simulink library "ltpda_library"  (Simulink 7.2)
settings: Solver=ode45  SolverMode=SingleTasking  StartTime=0.0  StopTime=10.0  RelTol=1e-3
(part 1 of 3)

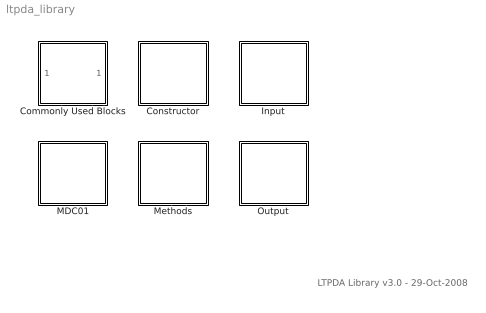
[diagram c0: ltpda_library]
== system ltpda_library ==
  note: LTPDA Library v3.0 - 29-Oct-2008
  Commonly Used Blocks : Subsystem
  Constructor : Subsystem  Tag=subsystem  AncestorBlock=libraryBase/SubSystName
  Input : Subsystem
  MDC01 : Subsystem  Tag=subsystem  AncestorBlock=libraryBase/SubSystName
  Methods : Subsystem  Tag=subsystem  AncestorBlock=libraryBase/SubSystName
  Output : Subsystem

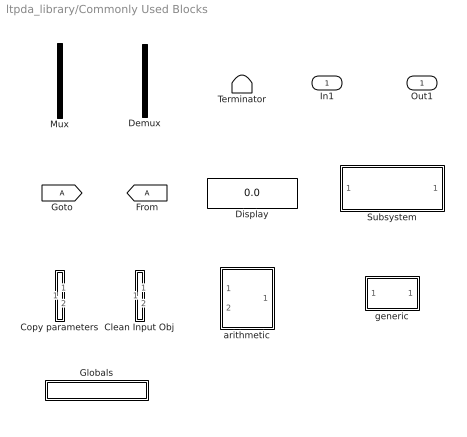
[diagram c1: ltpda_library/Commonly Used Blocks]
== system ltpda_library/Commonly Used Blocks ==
  In1 : Inport  OutDataType=sfix(16)  OutScaling=2^0
  Clean Input Obj : Subsystem
  Copy parameters : Subsystem
  Demux : Demux  Tag=demux  Outputs=2
  Display : Display
  Globals : Subsystem  Tag=globals
  Mux : Mux  Tag=mux  Inputs=2
  Subsystem : Subsystem
  Terminator : Terminator
  arithmetic : Subsystem  Tag=arithmetic
  generic : Subsystem  Tag=function
  Out1 : Outport  OutDataType=sfix(16)  OutScaling=2^0

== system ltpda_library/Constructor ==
  ltpda_getAOsInTimeSpan : Subsystem  Tag=function  AncestorBlock=libraryBase/function

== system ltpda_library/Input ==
  Object from list : Subsystem  Tag=input

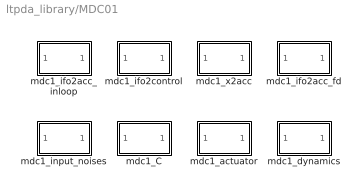
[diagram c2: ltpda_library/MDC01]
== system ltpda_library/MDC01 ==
  mdc1_C : Subsystem  Tag=function  AncestorBlock=libraryBase/function
  mdc1_actuator : Subsystem  Tag=function  AncestorBlock=libraryBase/function
  mdc1_dynamics : Subsystem  Tag=function  AncestorBlock=libraryBase/function
  mdc1_ifo2acc_fd : Subsystem  Tag=function  AncestorBlock=libraryBase/function
  mdc1_ifo2acc_inloop : Subsystem  Tag=function  AncestorBlock=libraryBase/function
  mdc1_ifo2control : Subsystem  Tag=function  AncestorBlock=libraryBase/function
  mdc1_input_noises : Subsystem  Tag=function  AncestorBlock=libraryBase/function
  mdc1_x2acc : Subsystem  Tag=function  AncestorBlock=libraryBase/function

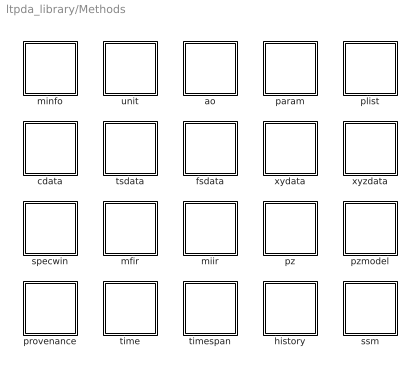
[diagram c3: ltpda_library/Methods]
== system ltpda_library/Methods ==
  ao : Subsystem  Tag=subsystem  AncestorBlock=libraryBase/SubSystName
  cdata : Subsystem  Tag=subsystem  AncestorBlock=libraryBase/SubSystName
  fsdata : Subsystem  Tag=subsystem  AncestorBlock=libraryBase/SubSystName
  history : Subsystem  Tag=subsystem  AncestorBlock=libraryBase/SubSystName
  mfir : Subsystem  Tag=subsystem  AncestorBlock=libraryBase/SubSystName
  miir : Subsystem  Tag=subsystem  AncestorBlock=libraryBase/SubSystName
  minfo : Subsystem  Tag=subsystem  AncestorBlock=libraryBase/SubSystName
  param : Subsystem  Tag=subsystem  AncestorBlock=libraryBase/SubSystName
  plist : Subsystem  Tag=subsystem  AncestorBlock=libraryBase/SubSystName
  provenance : Subsystem  Tag=subsystem  AncestorBlock=libraryBase/SubSystName
  pz : Subsystem  Tag=subsystem  AncestorBlock=libraryBase/SubSystName
  pzmodel : Subsystem  Tag=subsystem  AncestorBlock=libraryBase/SubSystName
  specwin : Subsystem  Tag=subsystem  AncestorBlock=libraryBase/SubSystName
  ssm : Subsystem  Tag=subsystem  AncestorBlock=libraryBase/SubSystName
  time : Subsystem  Tag=subsystem  AncestorBlock=libraryBase/SubSystName
  timespan : Subsystem  Tag=subsystem  AncestorBlock=libraryBase/SubSystName
  tsdata : Subsystem  Tag=subsystem  AncestorBlock=libraryBase/SubSystName
  unit : Subsystem  Tag=subsystem  AncestorBlock=libraryBase/SubSystName
  xydata : Subsystem  Tag=subsystem  AncestorBlock=libraryBase/SubSystName
  xyzdata : Subsystem  Tag=subsystem  AncestorBlock=libraryBase/SubSystName

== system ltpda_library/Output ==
  Send to output : Subsystem
  iplot : Subsystem  Tag=method ao
  plot : Subsystem  Tag=method ao
  save : Subsystem  Tag=method ao

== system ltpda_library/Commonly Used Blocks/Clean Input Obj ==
  In1 : Inport  OutDataType=sfix(16)  OutScaling=2^0
  In2 : Inport  Port=2  OutDataType=sfix(16)  OutScaling=2^0
  cleaninput : M-S-Function  FunctionName=g_cleaninput
  Out1 : Outport  OutDataType=sfix(16)  OutScaling=2^0
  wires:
  In2/1 -> cleaninput/2
  In1/1 -> cleaninput/1
  cleaninput/1 -> Out1/1

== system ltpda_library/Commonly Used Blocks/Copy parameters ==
  In1 : Inport  OutDataType=sfix(16)  OutScaling=2^0
  In2 : Inport  Port=2  OutDataType=sfix(16)  OutScaling=2^0
  copyparam : M-S-Function  FunctionName=g_copyparams
  Out1 : Outport  OutDataType=sfix(16)  OutScaling=2^0
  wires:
  copyparam/1 -> Out1/1
  In1/1 -> copyparam/1
  In2/1 -> copyparam/2

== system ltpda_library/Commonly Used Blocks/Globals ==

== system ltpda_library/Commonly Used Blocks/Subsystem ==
  In1 : Inport  OutDataType=sfix(16)  OutScaling=2^0
  Out1 : Outport  OutDataType=sfix(16)  OutScaling=2^0

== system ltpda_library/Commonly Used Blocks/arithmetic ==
  alpha : Inport  Tag=1  OutDataType=sfix(16)  OutScaling=2^0
  beta : Inport  Tag=2  Port=2  OutDataType=sfix(16)  OutScaling=2^0
  Mux : Mux  Tag=mux  Inputs=2
  arithmetic_func : M-S-Function  Tag=arithmetic  FunctionName=ltpdasim
  Out1 : Outport  OutDataType=sfix(16)  OutScaling=2^0
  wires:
  arithmetic_func/1 -> Out1/1
  Mux/1 -> arithmetic_func/1
  alpha/1 -> Mux/1
  beta/1 -> Mux/2

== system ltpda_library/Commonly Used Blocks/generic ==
  In1 : Inport  OutDataType=sfix(16)  OutScaling=2^0
  generic : M-S-Function  Tag=generic  FunctionName=ltpdasim
  Out1 : Outport  OutDataType=sfix(16)  OutScaling=2^0
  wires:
  generic/1 -> Out1/1
  In1/1 -> generic/1

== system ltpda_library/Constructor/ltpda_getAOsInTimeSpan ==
  In1 : Inport  OutDataType=sfix(16)  OutScaling=2^0
  ltpda_getAOsInTimeSpan : M-S-Function  Tag=ltpda_getAOsInTimeSpan  FunctionName=ltpdasim
  Out1 : Outport  OutDataType=sfix(16)  OutScaling=2^0
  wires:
  In1/1 -> ltpda_getAOsInTimeSpan/1
  ltpda_getAOsInTimeSpan/1 -> Out1/1

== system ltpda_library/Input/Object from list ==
  Input : Constant  Value=0  OutDataType=sfix(16)  OutScaling=2^0
  Input AO : Outport  OutDataType=sfix(16)  OutScaling=2^0
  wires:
  Input/1 -> Input AO/1

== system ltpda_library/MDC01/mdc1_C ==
  In1 : Inport  OutDataType=sfix(16)  OutScaling=2^0
  ltpda_mdc1_C : M-S-Function  Tag=ltpda_mdc1_C  FunctionName=ltpdasim
  Out1 : Outport  OutDataType=sfix(16)  OutScaling=2^0
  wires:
  In1/1 -> ltpda_mdc1_C/1
  ltpda_mdc1_C/1 -> Out1/1

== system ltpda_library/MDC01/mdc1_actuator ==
  In1 : Inport  OutDataType=sfix(16)  OutScaling=2^0
  ltpda_mdc1_actuator : M-S-Function  Tag=ltpda_mdc1_actuator  FunctionName=ltpdasim
  Out1 : Outport  OutDataType=sfix(16)  OutScaling=2^0
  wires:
  In1/1 -> ltpda_mdc1_actuator/1
  ltpda_mdc1_actuator/1 -> Out1/1

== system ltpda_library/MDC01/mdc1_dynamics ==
  In1 : Inport  OutDataType=sfix(16)  OutScaling=2^0
  ltpda_mdc1_dynamics : M-S-Function  Tag=ltpda_mdc1_dynamics  FunctionName=ltpdasim
  Out1 : Outport  OutDataType=sfix(16)  OutScaling=2^0
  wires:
  In1/1 -> ltpda_mdc1_dynamics/1
  ltpda_mdc1_dynamics/1 -> Out1/1

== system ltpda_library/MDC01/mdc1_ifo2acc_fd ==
  In1 : Inport  OutDataType=sfix(16)  OutScaling=2^0
  ltpda_mdc1_ifo2acc_fd : M-S-Function  Tag=ltpda_mdc1_ifo2acc_fd  FunctionName=ltpdasim
  Out1 : Outport  OutDataType=sfix(16)  OutScaling=2^0
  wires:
  In1/1 -> ltpda_mdc1_ifo2acc_fd/1
  ltpda_mdc1_ifo2acc_fd/1 -> Out1/1

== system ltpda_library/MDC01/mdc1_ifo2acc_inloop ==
  In1 : Inport  OutDataType=sfix(16)  OutScaling=2^0
  ltpda_mdc1_ifo2acc_inloop : M-S-Function  Tag=ltpda_mdc1_ifo2acc_inloop  FunctionName=ltpdasim
  Out1 : Outport  OutDataType=sfix(16)  OutScaling=2^0
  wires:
  In1/1 -> ltpda_mdc1_ifo2acc_inloop/1
  ltpda_mdc1_ifo2acc_inloop/1 -> Out1/1

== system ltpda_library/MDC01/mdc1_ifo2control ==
  In1 : Inport  OutDataType=sfix(16)  OutScaling=2^0
  ltpda_mdc1_ifo2control : M-S-Function  Tag=ltpda_mdc1_ifo2control  FunctionName=ltpdasim
  Out1 : Outport  OutDataType=sfix(16)  OutScaling=2^0
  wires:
  In1/1 -> ltpda_mdc1_ifo2control/1
  ltpda_mdc1_ifo2control/1 -> Out1/1

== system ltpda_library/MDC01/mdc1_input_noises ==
  In1 : Inport  OutDataType=sfix(16)  OutScaling=2^0
  ltpda_mdc1_input_noises : M-S-Function  Tag=ltpda_mdc1_input_noises  FunctionName=ltpdasim
  Out1 : Outport  OutDataType=sfix(16)  OutScaling=2^0
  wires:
  In1/1 -> ltpda_mdc1_input_noises/1
  ltpda_mdc1_input_noises/1 -> Out1/1

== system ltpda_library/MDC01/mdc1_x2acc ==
  In1 : Inport  OutDataType=sfix(16)  OutScaling=2^0
  ltpda_mdc1_x2acc : M-S-Function  Tag=ltpda_mdc1_x2acc  FunctionName=ltpdasim
  Out1 : Outport  OutDataType=sfix(16)  OutScaling=2^0
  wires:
  In1/1 -> ltpda_mdc1_x2acc/1
  ltpda_mdc1_x2acc/1 -> Out1/1

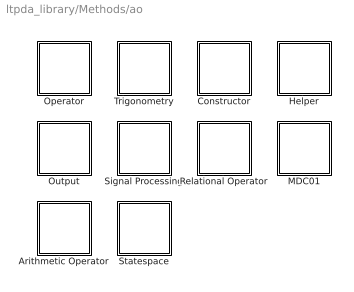
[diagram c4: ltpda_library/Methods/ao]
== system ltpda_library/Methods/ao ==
  Arithmetic Operator : Subsystem  Tag=subsystem  AncestorBlock=libraryBase/SubSystName
  Constructor : Subsystem  Tag=subsystem  AncestorBlock=libraryBase/SubSystName
  Helper : Subsystem  Tag=subsystem  AncestorBlock=libraryBase/SubSystName
  MDC01 : Subsystem  Tag=subsystem  AncestorBlock=libraryBase/SubSystName
  Operator : Subsystem  Tag=subsystem  AncestorBlock=libraryBase/SubSystName
  Output : Subsystem  Tag=subsystem  AncestorBlock=libraryBase/SubSystName
  Relational Operator : Subsystem  Tag=subsystem  AncestorBlock=libraryBase/SubSystName
  Signal Processing : Subsystem  Tag=subsystem  AncestorBlock=libraryBase/SubSystName
  Statespace : Subsystem  Tag=subsystem  AncestorBlock=libraryBase/SubSystName
  Trigonometry : Subsystem  Tag=subsystem  AncestorBlock=libraryBase/SubSystName

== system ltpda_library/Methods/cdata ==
  Constructor : Subsystem  Tag=subsystem  AncestorBlock=libraryBase/SubSystName
  Helper : Subsystem  Tag=subsystem  AncestorBlock=libraryBase/SubSystName
  Output : Subsystem  Tag=subsystem  AncestorBlock=libraryBase/SubSystName
  Relational Operator : Subsystem  Tag=subsystem  AncestorBlock=libraryBase/SubSystName

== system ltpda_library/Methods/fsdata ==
  Constructor : Subsystem  Tag=subsystem  AncestorBlock=libraryBase/SubSystName
  Helper : Subsystem  Tag=subsystem  AncestorBlock=libraryBase/SubSystName
  Output : Subsystem  Tag=subsystem  AncestorBlock=libraryBase/SubSystName
  Relational Operator : Subsystem  Tag=subsystem  AncestorBlock=libraryBase/SubSystName

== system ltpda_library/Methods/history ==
  Constructor : Subsystem  Tag=subsystem  AncestorBlock=libraryBase/SubSystName
  Helper : Subsystem  Tag=subsystem  AncestorBlock=libraryBase/SubSystName
  Output : Subsystem  Tag=subsystem  AncestorBlock=libraryBase/SubSystName
  Relational Operator : Subsystem  Tag=subsystem  AncestorBlock=libraryBase/SubSystName

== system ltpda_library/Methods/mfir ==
  Constructor : Subsystem  Tag=subsystem  AncestorBlock=libraryBase/SubSystName
  Helper : Subsystem  Tag=subsystem  AncestorBlock=libraryBase/SubSystName
  Output : Subsystem  Tag=subsystem  AncestorBlock=libraryBase/SubSystName
  Relational Operator : Subsystem  Tag=subsystem  AncestorBlock=libraryBase/SubSystName
  Signal Processing : Subsystem  Tag=subsystem  AncestorBlock=libraryBase/SubSystName
  Statespace : Subsystem  Tag=subsystem  AncestorBlock=libraryBase/SubSystName

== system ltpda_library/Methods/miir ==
  Constructor : Subsystem  Tag=subsystem  AncestorBlock=libraryBase/SubSystName
  Helper : Subsystem  Tag=subsystem  AncestorBlock=libraryBase/SubSystName
  Output : Subsystem  Tag=subsystem  AncestorBlock=libraryBase/SubSystName
  Relational Operator : Subsystem  Tag=subsystem  AncestorBlock=libraryBase/SubSystName
  Signal Processing : Subsystem  Tag=subsystem  AncestorBlock=libraryBase/SubSystName
  Statespace : Subsystem  Tag=subsystem  AncestorBlock=libraryBase/SubSystName

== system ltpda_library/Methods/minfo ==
  Constructor : Subsystem  Tag=subsystem  AncestorBlock=libraryBase/SubSystName
  Helper : Subsystem  Tag=subsystem  AncestorBlock=libraryBase/SubSystName
  Output : Subsystem  Tag=subsystem  AncestorBlock=libraryBase/SubSystName
  Relational Operator : Subsystem  Tag=subsystem  AncestorBlock=libraryBase/SubSystName

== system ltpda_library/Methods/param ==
  Constructor : Subsystem  Tag=subsystem  AncestorBlock=libraryBase/SubSystName
  Helper : Subsystem  Tag=subsystem  AncestorBlock=libraryBase/SubSystName
  Output : Subsystem  Tag=subsystem  AncestorBlock=libraryBase/SubSystName
  Relational Operator : Subsystem  Tag=subsystem  AncestorBlock=libraryBase/SubSystName

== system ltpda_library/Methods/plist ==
  Constructor : Subsystem  Tag=subsystem  AncestorBlock=libraryBase/SubSystName
  Helper : Subsystem  Tag=subsystem  AncestorBlock=libraryBase/SubSystName
  Output : Subsystem  Tag=subsystem  AncestorBlock=libraryBase/SubSystName
  Relational Operator : Subsystem  Tag=subsystem  AncestorBlock=libraryBase/SubSystName
  Signal Processing : Subsystem  Tag=subsystem  AncestorBlock=libraryBase/SubSystName

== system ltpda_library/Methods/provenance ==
  Constructor : Subsystem  Tag=subsystem  AncestorBlock=libraryBase/SubSystName
  Helper : Subsystem  Tag=subsystem  AncestorBlock=libraryBase/SubSystName
  Output : Subsystem  Tag=subsystem  AncestorBlock=libraryBase/SubSystName
  Relational Operator : Subsystem  Tag=subsystem  AncestorBlock=libraryBase/SubSystName

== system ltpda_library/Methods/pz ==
  Constructor : Subsystem  Tag=subsystem  AncestorBlock=libraryBase/SubSystName
  Helper : Subsystem  Tag=subsystem  AncestorBlock=libraryBase/SubSystName
  Output : Subsystem  Tag=subsystem  AncestorBlock=libraryBase/SubSystName
  Relational Operator : Subsystem  Tag=subsystem  AncestorBlock=libraryBase/SubSystName
  Signal Processing : Subsystem  Tag=subsystem  AncestorBlock=libraryBase/SubSystName

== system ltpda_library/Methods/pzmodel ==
  Constructor : Subsystem  Tag=subsystem  AncestorBlock=libraryBase/SubSystName
  Helper : Subsystem  Tag=subsystem  AncestorBlock=libraryBase/SubSystName
  Operator : Subsystem  Tag=subsystem  AncestorBlock=libraryBase/SubSystName
  Output : Subsystem  Tag=subsystem  AncestorBlock=libraryBase/SubSystName
  Relational Operator : Subsystem  Tag=subsystem  AncestorBlock=libraryBase/SubSystName
  Signal Processing : Subsystem  Tag=subsystem  AncestorBlock=libraryBase/SubSystName
  Statespace : Subsystem  Tag=subsystem  AncestorBlock=libraryBase/SubSystName

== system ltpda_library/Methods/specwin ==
  Constructor : Subsystem  Tag=subsystem  AncestorBlock=libraryBase/SubSystName
  Helper : Subsystem  Tag=subsystem  AncestorBlock=libraryBase/SubSystName
  Output : Subsystem  Tag=subsystem  AncestorBlock=libraryBase/SubSystName
  Relational Operator : Subsystem  Tag=subsystem  AncestorBlock=libraryBase/SubSystName

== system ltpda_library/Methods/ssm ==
  Constructor : Subsystem  Tag=subsystem  AncestorBlock=libraryBase/SubSystName
  Helper : Subsystem  Tag=subsystem  AncestorBlock=libraryBase/SubSystName
  Output : Subsystem  Tag=subsystem  AncestorBlock=libraryBase/SubSystName
  Relational Operator : Subsystem  Tag=subsystem  AncestorBlock=libraryBase/SubSystName
  STATESPACE : Subsystem  Tag=subsystem  AncestorBlock=libraryBase/SubSystName
  Statespace : Subsystem  Tag=subsystem  AncestorBlock=libraryBase/SubSystName

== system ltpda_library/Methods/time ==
  Arithmetic Operator : Subsystem  Tag=subsystem  AncestorBlock=libraryBase/SubSystName
  Constructor : Subsystem  Tag=subsystem  AncestorBlock=libraryBase/SubSystName
  Helper : Subsystem  Tag=subsystem  AncestorBlock=libraryBase/SubSystName
  Output : Subsystem  Tag=subsystem  AncestorBlock=libraryBase/SubSystName
  Relational Operator : Subsystem  Tag=subsystem  AncestorBlock=libraryBase/SubSystName

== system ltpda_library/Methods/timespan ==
  Constructor : Subsystem  Tag=subsystem  AncestorBlock=libraryBase/SubSystName
  Helper : Subsystem  Tag=subsystem  AncestorBlock=libraryBase/SubSystName
  Output : Subsystem  Tag=subsystem  AncestorBlock=libraryBase/SubSystName
  Relational Operator : Subsystem  Tag=subsystem  AncestorBlock=libraryBase/SubSystName
  Statespace : Subsystem  Tag=subsystem  AncestorBlock=libraryBase/SubSystName

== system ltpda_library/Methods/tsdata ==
  Constructor : Subsystem  Tag=subsystem  AncestorBlock=libraryBase/SubSystName
  Helper : Subsystem  Tag=subsystem  AncestorBlock=libraryBase/SubSystName
  Output : Subsystem  Tag=subsystem  AncestorBlock=libraryBase/SubSystName
  Relational Operator : Subsystem  Tag=subsystem  AncestorBlock=libraryBase/SubSystName

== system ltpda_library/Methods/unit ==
  Constructor : Subsystem  Tag=subsystem  AncestorBlock=libraryBase/SubSystName
  Helper : Subsystem  Tag=subsystem  AncestorBlock=libraryBase/SubSystName
  Output : Subsystem  Tag=subsystem  AncestorBlock=libraryBase/SubSystName
  Relational Operator : Subsystem  Tag=subsystem  AncestorBlock=libraryBase/SubSystName

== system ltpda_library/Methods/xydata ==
  Constructor : Subsystem  Tag=subsystem  AncestorBlock=libraryBase/SubSystName
  Helper : Subsystem  Tag=subsystem  AncestorBlock=libraryBase/SubSystName
  Output : Subsystem  Tag=subsystem  AncestorBlock=libraryBase/SubSystName
  Relational Operator : Subsystem  Tag=subsystem  AncestorBlock=libraryBase/SubSystName

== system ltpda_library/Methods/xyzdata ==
  Constructor : Subsystem  Tag=subsystem  AncestorBlock=libraryBase/SubSystName
  Helper : Subsystem  Tag=subsystem  AncestorBlock=libraryBase/SubSystName
  Output : Subsystem  Tag=subsystem  AncestorBlock=libraryBase/SubSystName
  Relational Operator : Subsystem  Tag=subsystem  AncestorBlock=libraryBase/SubSystName

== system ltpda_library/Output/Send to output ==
  In1 : Inport  OutDataType=sfix(16)  OutScaling=2^0
  save result : M-S-Function  FunctionName=g_saveresult
  Out1 : Outport  OutDataType=sfix(16)  OutScaling=2^0
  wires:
  In1/1 -> save result/1
  save result/1 -> Out1/1

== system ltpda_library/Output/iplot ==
  In1 : Inport  OutDataType=sfix(16)  OutScaling=2^0
  Terminator : Terminator
  iplot : M-S-Function  Tag=iplot  FunctionName=ltpdasim
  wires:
  In1/1 -> iplot/1
  iplot/1 -> Terminator/1

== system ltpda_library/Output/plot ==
  In1 : Inport  OutDataType=sfix(16)  OutScaling=2^0
  Terminator : Terminator
  plot : M-S-Function  Tag=plot  FunctionName=ltpdasim
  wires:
  In1/1 -> plot/1
  plot/1 -> Terminator/1

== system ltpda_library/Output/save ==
  In1 : Inport  OutDataType=sfix(16)  OutScaling=2^0
  Terminator : Terminator
  save : M-S-Function  Tag=save  FunctionName=ltpdasim
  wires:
  In1/1 -> save/1
  save/1 -> Terminator/1

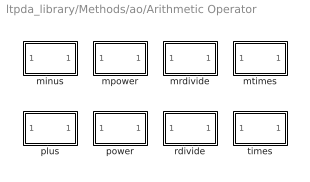
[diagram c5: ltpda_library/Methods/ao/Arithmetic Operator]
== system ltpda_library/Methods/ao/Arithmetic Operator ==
  minus : Subsystem  Tag=method ao  AncestorBlock=libraryBase/function
  mpower : Subsystem  Tag=method ao  AncestorBlock=libraryBase/function
  mrdivide : Subsystem  Tag=method ao  AncestorBlock=libraryBase/function
  mtimes : Subsystem  Tag=method ao  AncestorBlock=libraryBase/function
  plus : Subsystem  Tag=method ao  AncestorBlock=libraryBase/function
  power : Subsystem  Tag=method ao  AncestorBlock=libraryBase/function
  rdivide : Subsystem  Tag=method ao  AncestorBlock=libraryBase/function
  times : Subsystem  Tag=method ao  AncestorBlock=libraryBase/function

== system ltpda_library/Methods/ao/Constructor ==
  ao : Subsystem  Tag=method ao  AncestorBlock=libraryBase/constructor
  rebuild : Subsystem  Tag=method ao  AncestorBlock=libraryBase/constructor

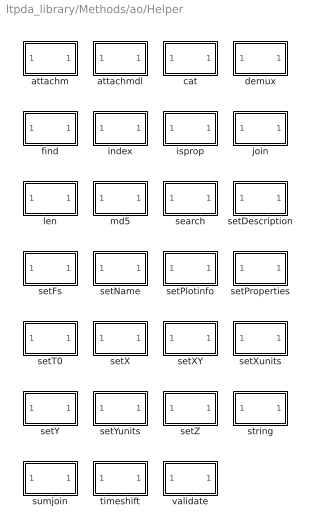
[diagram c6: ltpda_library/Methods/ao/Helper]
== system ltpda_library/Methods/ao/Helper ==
  attachm : Subsystem  Tag=method ao  AncestorBlock=libraryBase/function
  attachmdl : Subsystem  Tag=method ao  AncestorBlock=libraryBase/function
  cat : Subsystem  Tag=method ao  AncestorBlock=libraryBase/function
  demux : Subsystem  Tag=method ao  AncestorBlock=libraryBase/function
  find : Subsystem  Tag=method ao  AncestorBlock=libraryBase/function
  index : Subsystem  Tag=method ao  AncestorBlock=libraryBase/function
  isprop : Subsystem  Tag=method ao  AncestorBlock=libraryBase/function
  join : Subsystem  Tag=method ao  AncestorBlock=libraryBase/function
  len : Subsystem  Tag=method ao  AncestorBlock=libraryBase/function
  md5 : Subsystem  Tag=method ao  AncestorBlock=libraryBase/function
  search : Subsystem  Tag=method ao  AncestorBlock=libraryBase/function
  setDescription : Subsystem  Tag=method ao  AncestorBlock=libraryBase/function
  setFs : Subsystem  Tag=method ao  AncestorBlock=libraryBase/function
  setName : Subsystem  Tag=method ao  AncestorBlock=libraryBase/function
  setPlotinfo : Subsystem  Tag=method ao  AncestorBlock=libraryBase/function
  setProperties : Subsystem  Tag=method ao  AncestorBlock=libraryBase/function
  setT0 : Subsystem  Tag=method ao  AncestorBlock=libraryBase/function
  setX : Subsystem  Tag=method ao  AncestorBlock=libraryBase/function
  setXY : Subsystem  Tag=method ao  AncestorBlock=libraryBase/function
  setXunits : Subsystem  Tag=method ao  AncestorBlock=libraryBase/function
  setY : Subsystem  Tag=method ao  AncestorBlock=libraryBase/function
  setYunits : Subsystem  Tag=method ao  AncestorBlock=libraryBase/function
  setZ : Subsystem  Tag=method ao  AncestorBlock=libraryBase/function
  string : Subsystem  Tag=method ao  AncestorBlock=libraryBase/function
  sumjoin : Subsystem  Tag=method ao  AncestorBlock=libraryBase/function
  timeshift : Subsystem  Tag=method ao  AncestorBlock=libraryBase/function
  validate : Subsystem  Tag=method ao  AncestorBlock=libraryBase/function

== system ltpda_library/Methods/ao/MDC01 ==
  mdc1_ifo2acc_fd : Subsystem  Tag=method ao  AncestorBlock=libraryBase/function
  mdc1_ifo2acc_inloop : Subsystem  Tag=method ao  AncestorBlock=libraryBase/function
  mdc1_ifo2control : Subsystem  Tag=method ao  AncestorBlock=libraryBase/function
  mdc1_x2acc : Subsystem  Tag=method ao  AncestorBlock=libraryBase/function

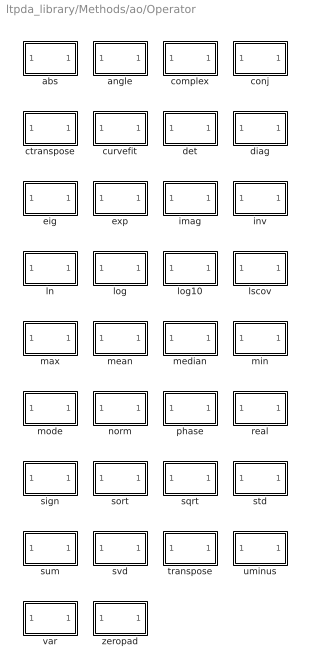
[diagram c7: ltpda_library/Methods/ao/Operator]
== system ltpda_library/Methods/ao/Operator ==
  abs : Subsystem  Tag=method ao  AncestorBlock=libraryBase/function
  angle : Subsystem  Tag=method ao  AncestorBlock=libraryBase/function
  complex : Subsystem  Tag=method ao  AncestorBlock=libraryBase/function
  conj : Subsystem  Tag=method ao  AncestorBlock=libraryBase/function
  ctranspose : Subsystem  Tag=method ao  AncestorBlock=libraryBase/function
  curvefit : Subsystem  Tag=method ao  AncestorBlock=libraryBase/function
  det : Subsystem  Tag=method ao  AncestorBlock=libraryBase/function
  diag : Subsystem  Tag=method ao  AncestorBlock=libraryBase/function
  eig : Subsystem  Tag=method ao  AncestorBlock=libraryBase/function
  exp : Subsystem  Tag=method ao  AncestorBlock=libraryBase/function
  imag : Subsystem  Tag=method ao  AncestorBlock=libraryBase/function
  inv : Subsystem  Tag=method ao  AncestorBlock=libraryBase/function
  ln : Subsystem  Tag=method ao  AncestorBlock=libraryBase/function
  log : Subsystem  Tag=method ao  AncestorBlock=libraryBase/function
  log10 : Subsystem  Tag=method ao  AncestorBlock=libraryBase/function
  lscov : Subsystem  Tag=method ao  AncestorBlock=libraryBase/function
  max : Subsystem  Tag=method ao  AncestorBlock=libraryBase/function
  mean : Subsystem  Tag=method ao  AncestorBlock=libraryBase/function
  median : Subsystem  Tag=method ao  AncestorBlock=libraryBase/function
  min : Subsystem  Tag=method ao  AncestorBlock=libraryBase/function
  mode : Subsystem  Tag=method ao  AncestorBlock=libraryBase/function
  norm : Subsystem  Tag=method ao  AncestorBlock=libraryBase/function
  phase : Subsystem  Tag=method ao  AncestorBlock=libraryBase/function
  real : Subsystem  Tag=method ao  AncestorBlock=libraryBase/function
  sign : Subsystem  Tag=method ao  AncestorBlock=libraryBase/function
  sort : Subsystem  Tag=method ao  AncestorBlock=libraryBase/function
  sqrt : Subsystem  Tag=method ao  AncestorBlock=libraryBase/function
  std : Subsystem  Tag=method ao  AncestorBlock=libraryBase/function
  sum : Subsystem  Tag=method ao  AncestorBlock=libraryBase/function
  svd : Subsystem  Tag=method ao  AncestorBlock=libraryBase/function
  transpose : Subsystem  Tag=method ao  AncestorBlock=libraryBase/function
  uminus : Subsystem  Tag=method ao  AncestorBlock=libraryBase/function
  var : Subsystem  Tag=method ao  AncestorBlock=libraryBase/function
  zeropad : Subsystem  Tag=method ao  AncestorBlock=libraryBase/function

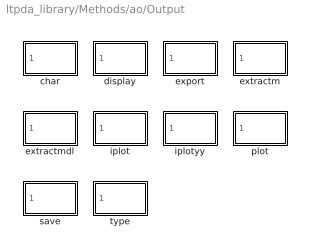
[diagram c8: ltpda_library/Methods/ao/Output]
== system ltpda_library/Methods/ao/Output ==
  char : Subsystem  Tag=method ao  AncestorBlock=libraryBase/output
  display : Subsystem  Tag=method ao  AncestorBlock=libraryBase/output
  export : Subsystem  Tag=method ao  AncestorBlock=libraryBase/output
  extractm : Subsystem  Tag=method ao  AncestorBlock=libraryBase/output
  extractmdl : Subsystem  Tag=method ao  AncestorBlock=libraryBase/output
  iplot : Subsystem  Tag=method ao  AncestorBlock=libraryBase/output
  iplotyy : Subsystem  Tag=method ao  AncestorBlock=libraryBase/output
  plot : Subsystem  Tag=method ao  AncestorBlock=libraryBase/output
  save : Subsystem  Tag=method ao  AncestorBlock=libraryBase/output
  type : Subsystem  Tag=method ao  AncestorBlock=libraryBase/output

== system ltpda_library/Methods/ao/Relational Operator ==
  eq : Subsystem  Tag=method ao  AncestorBlock=libraryBase/function
  ge : Subsystem  Tag=method ao  AncestorBlock=libraryBase/function
  gt : Subsystem  Tag=method ao  AncestorBlock=libraryBase/function
  le : Subsystem  Tag=method ao  AncestorBlock=libraryBase/function
  lt : Subsystem  Tag=method ao  AncestorBlock=libraryBase/function
  ne : Subsystem  Tag=method ao  AncestorBlock=libraryBase/function

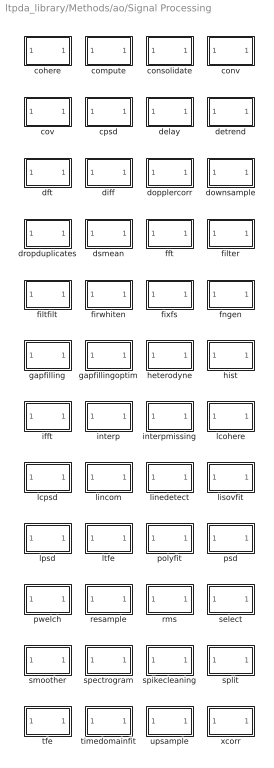
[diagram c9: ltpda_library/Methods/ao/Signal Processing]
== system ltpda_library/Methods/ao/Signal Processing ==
  cohere : Subsystem  Tag=method ao  AncestorBlock=libraryBase/function
  compute : Subsystem  Tag=method ao  AncestorBlock=libraryBase/function
  consolidate : Subsystem  Tag=method ao  AncestorBlock=libraryBase/function
  conv : Subsystem  Tag=method ao  AncestorBlock=libraryBase/function
  cov : Subsystem  Tag=method ao  AncestorBlock=libraryBase/function
  cpsd : Subsystem  Tag=method ao  AncestorBlock=libraryBase/function
  delay : Subsystem  Tag=method ao  AncestorBlock=libraryBase/function
  detrend : Subsystem  Tag=method ao  AncestorBlock=libraryBase/function
  dft : Subsystem  Tag=method ao  AncestorBlock=libraryBase/function
  diff : Subsystem  Tag=method ao  AncestorBlock=libraryBase/function
  dopplercorr : Subsystem  Tag=method ao  AncestorBlock=libraryBase/function
  downsample : Subsystem  Tag=method ao  AncestorBlock=libraryBase/function
  dropduplicates : Subsystem  Tag=method ao  AncestorBlock=libraryBase/function
  dsmean : Subsystem  Tag=method ao  AncestorBlock=libraryBase/function
  fft : Subsystem  Tag=method ao  AncestorBlock=libraryBase/function
  filter : Subsystem  Tag=method ao  AncestorBlock=libraryBase/function
  filtfilt : Subsystem  Tag=method ao  AncestorBlock=libraryBase/function
  firwhiten : Subsystem  Tag=method ao  AncestorBlock=libraryBase/function
  fixfs : Subsystem  Tag=method ao  AncestorBlock=libraryBase/function
  fngen : Subsystem  Tag=method ao  AncestorBlock=libraryBase/function
  gapfilling : Subsystem  Tag=method ao  AncestorBlock=libraryBase/function
  gapfillingoptim : Subsystem  Tag=method ao  AncestorBlock=libraryBase/function
  heterodyne : Subsystem  Tag=method ao  AncestorBlock=libraryBase/function
  hist : Subsystem  Tag=method ao  AncestorBlock=libraryBase/function
  ifft : Subsystem  Tag=method ao  AncestorBlock=libraryBase/function
  interp : Subsystem  Tag=method ao  AncestorBlock=libraryBase/function
  interpmissing : Subsystem  Tag=method ao  AncestorBlock=libraryBase/function
  lcohere : Subsystem  Tag=method ao  AncestorBlock=libraryBase/function
  lcpsd : Subsystem  Tag=method ao  AncestorBlock=libraryBase/function
  lincom : Subsystem  Tag=method ao  AncestorBlock=libraryBase/function
  linedetect : Subsystem  Tag=method ao  AncestorBlock=libraryBase/function
  lisovfit : Subsystem  Tag=method ao  AncestorBlock=libraryBase/function
  lpsd : Subsystem  Tag=method ao  AncestorBlock=libraryBase/function
  ltfe : Subsystem  Tag=method ao  AncestorBlock=libraryBase/function
  polyfit : Subsystem  Tag=method ao  AncestorBlock=libraryBase/function
  psd : Subsystem  Tag=method ao  AncestorBlock=libraryBase/function
  pwelch : Subsystem  Tag=method ao  AncestorBlock=libraryBase/function
  resample : Subsystem  Tag=method ao  AncestorBlock=libraryBase/function
  rms : Subsystem  Tag=method ao  AncestorBlock=libraryBase/function
  select : Subsystem  Tag=method ao  AncestorBlock=libraryBase/function
  smoother : Subsystem  Tag=method ao  AncestorBlock=libraryBase/function
  spectrogram : Subsystem  Tag=method ao  AncestorBlock=libraryBase/function
  spikecleaning : Subsystem  Tag=method ao  AncestorBlock=libraryBase/function
  split : Subsystem  Tag=method ao  AncestorBlock=libraryBase/function
  tfe : Subsystem  Tag=method ao  AncestorBlock=libraryBase/function
  timedomainfit : Subsystem  Tag=method ao  AncestorBlock=libraryBase/function
  upsample : Subsystem  Tag=method ao  AncestorBlock=libraryBase/function
  xcorr : Subsystem  Tag=method ao  AncestorBlock=libraryBase/function

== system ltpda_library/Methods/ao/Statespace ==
  report : Subsystem  Tag=method ao  AncestorBlock=libraryBase/function

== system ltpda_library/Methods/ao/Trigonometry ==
  acos : Subsystem  Tag=method ao  AncestorBlock=libraryBase/function
  asin : Subsystem  Tag=method ao  AncestorBlock=libraryBase/function
  atan : Subsystem  Tag=method ao  AncestorBlock=libraryBase/function
  atan2 : Subsystem  Tag=method ao  AncestorBlock=libraryBase/function
  cos : Subsystem  Tag=method ao  AncestorBlock=libraryBase/function
  sin : Subsystem  Tag=method ao  AncestorBlock=libraryBase/function
  tan : Subsystem  Tag=method ao  AncestorBlock=libraryBase/function

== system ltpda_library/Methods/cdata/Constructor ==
  cdata : Subsystem  Tag=method cdata  AncestorBlock=libraryBase/constructor

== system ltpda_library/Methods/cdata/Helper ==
  isprop : Subsystem  Tag=method cdata  AncestorBlock=libraryBase/function

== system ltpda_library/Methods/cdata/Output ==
  display : Subsystem  Tag=method cdata  AncestorBlock=libraryBase/output

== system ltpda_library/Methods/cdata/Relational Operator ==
  eq : Subsystem  Tag=method cdata  AncestorBlock=libraryBase/function
  ne : Subsystem  Tag=method cdata  AncestorBlock=libraryBase/function

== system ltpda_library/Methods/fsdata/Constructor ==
  fsdata : Subsystem  Tag=method fsdata  AncestorBlock=libraryBase/constructor

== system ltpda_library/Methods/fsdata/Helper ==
  isprop : Subsystem  Tag=method fsdata  AncestorBlock=libraryBase/function

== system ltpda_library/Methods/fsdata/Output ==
  char : Subsystem  Tag=method fsdata  AncestorBlock=libraryBase/output
  display : Subsystem  Tag=method fsdata  AncestorBlock=libraryBase/output

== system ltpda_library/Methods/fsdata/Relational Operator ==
  eq : Subsystem  Tag=method fsdata  AncestorBlock=libraryBase/function
  ne : Subsystem  Tag=method fsdata  AncestorBlock=libraryBase/function

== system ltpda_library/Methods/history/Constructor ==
  history : Subsystem  Tag=method history  AncestorBlock=libraryBase/constructor
  rebuild : Subsystem  Tag=method history  AncestorBlock=libraryBase/constructor

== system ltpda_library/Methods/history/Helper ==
  isprop : Subsystem  Tag=method history  AncestorBlock=libraryBase/function

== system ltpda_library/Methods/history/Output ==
  char : Subsystem  Tag=method history  AncestorBlock=libraryBase/output
  display : Subsystem  Tag=method history  AncestorBlock=libraryBase/output
  dotview : Subsystem  Tag=method history  AncestorBlock=libraryBase/output
  hist2dot : Subsystem  Tag=method history  AncestorBlock=libraryBase/output
  hist2m : Subsystem  Tag=method history  AncestorBlock=libraryBase/output
  plot : Subsystem  Tag=method history  AncestorBlock=libraryBase/output
  string : Subsystem  Tag=method history  AncestorBlock=libraryBase/output

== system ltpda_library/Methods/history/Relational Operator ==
  eq : Subsystem  Tag=method history  AncestorBlock=libraryBase/function
  ne : Subsystem  Tag=method history  AncestorBlock=libraryBase/function

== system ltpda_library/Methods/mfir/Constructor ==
  mfir : Subsystem  Tag=method mfir  AncestorBlock=libraryBase/constructor
  rebuild : Subsystem  Tag=method mfir  AncestorBlock=libraryBase/constructor

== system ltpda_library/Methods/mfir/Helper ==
  isprop : Subsystem  Tag=method mfir  AncestorBlock=libraryBase/function
  redesign : Subsystem  Tag=method mfir  AncestorBlock=libraryBase/function
  setIunits : Subsystem  Tag=method mfir  AncestorBlock=libraryBase/function
  setName : Subsystem  Tag=method mfir  AncestorBlock=libraryBase/function
  setOunits : Subsystem  Tag=method mfir  AncestorBlock=libraryBase/function
  setProperties : Subsystem  Tag=method mfir  AncestorBlock=libraryBase/function

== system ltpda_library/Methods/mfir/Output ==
  char : Subsystem  Tag=method mfir  AncestorBlock=libraryBase/output
  display : Subsystem  Tag=method mfir  AncestorBlock=libraryBase/output
  save : Subsystem  Tag=method mfir  AncestorBlock=libraryBase/output
  string : Subsystem  Tag=method mfir  AncestorBlock=libraryBase/output
  type : Subsystem  Tag=method mfir  AncestorBlock=libraryBase/output

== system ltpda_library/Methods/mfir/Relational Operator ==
  eq : Subsystem  Tag=method mfir  AncestorBlock=libraryBase/function
  ne : Subsystem  Tag=method mfir  AncestorBlock=libraryBase/function

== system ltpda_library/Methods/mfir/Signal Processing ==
  oldresp : Subsystem  Tag=method mfir  AncestorBlock=libraryBase/function
  resp : Subsystem  Tag=method mfir  AncestorBlock=libraryBase/function

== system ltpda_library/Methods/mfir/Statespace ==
  report : Subsystem  Tag=method mfir  AncestorBlock=libraryBase/function

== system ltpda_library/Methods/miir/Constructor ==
  miir : Subsystem  Tag=method miir  AncestorBlock=libraryBase/constructor
  rebuild : Subsystem  Tag=method miir  AncestorBlock=libraryBase/constructor

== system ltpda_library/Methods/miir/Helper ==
  isprop : Subsystem  Tag=method miir  AncestorBlock=libraryBase/function
  redesign : Subsystem  Tag=method miir  AncestorBlock=libraryBase/function
  setIunits : Subsystem  Tag=method miir  AncestorBlock=libraryBase/function
  setName : Subsystem  Tag=method miir  AncestorBlock=libraryBase/function
  setOunits : Subsystem  Tag=method miir  AncestorBlock=libraryBase/function
  setProperties : Subsystem  Tag=method miir  AncestorBlock=libraryBase/function

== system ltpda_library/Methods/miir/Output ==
  char : Subsystem  Tag=method miir  AncestorBlock=libraryBase/output
  display : Subsystem  Tag=method miir  AncestorBlock=libraryBase/output
  save : Subsystem  Tag=method miir  AncestorBlock=libraryBase/output
  string : Subsystem  Tag=method miir  AncestorBlock=libraryBase/output
  type : Subsystem  Tag=method miir  AncestorBlock=libraryBase/output

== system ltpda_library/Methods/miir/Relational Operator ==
  eq : Subsystem  Tag=method miir  AncestorBlock=libraryBase/function
  ne : Subsystem  Tag=method miir  AncestorBlock=libraryBase/function

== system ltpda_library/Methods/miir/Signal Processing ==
  oldresp : Subsystem  Tag=method miir  AncestorBlock=libraryBase/function
  resp : Subsystem  Tag=method miir  AncestorBlock=libraryBase/function

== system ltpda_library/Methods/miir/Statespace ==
  report : Subsystem  Tag=method miir  AncestorBlock=libraryBase/function

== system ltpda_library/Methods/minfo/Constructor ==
  minfo : Subsystem  Tag=method minfo  AncestorBlock=libraryBase/constructor

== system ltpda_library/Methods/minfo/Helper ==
  isprop : Subsystem  Tag=method minfo  AncestorBlock=libraryBase/function

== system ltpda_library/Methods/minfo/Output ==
  char : Subsystem  Tag=method minfo  AncestorBlock=libraryBase/output
  display : Subsystem  Tag=method minfo  AncestorBlock=libraryBase/output

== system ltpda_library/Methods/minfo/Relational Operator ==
  eq : Subsystem  Tag=method minfo  AncestorBlock=libraryBase/function
  ne : Subsystem  Tag=method minfo  AncestorBlock=libraryBase/function

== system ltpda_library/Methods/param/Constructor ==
  param : Subsystem  Tag=method param  AncestorBlock=libraryBase/constructor

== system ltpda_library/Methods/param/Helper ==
  isprop : Subsystem  Tag=method param  AncestorBlock=libraryBase/function
  mux : Subsystem  Tag=method param  AncestorBlock=libraryBase/function

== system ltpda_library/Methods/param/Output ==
  char : Subsystem  Tag=method param  AncestorBlock=libraryBase/output
  display : Subsystem  Tag=method param  AncestorBlock=libraryBase/output
  string : Subsystem  Tag=method param  AncestorBlock=libraryBase/output

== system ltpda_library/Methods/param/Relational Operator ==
  eq : Subsystem  Tag=method param  AncestorBlock=libraryBase/function
  ne : Subsystem  Tag=method param  AncestorBlock=libraryBase/function

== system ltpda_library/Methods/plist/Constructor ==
  plist : Subsystem  Tag=method plist  AncestorBlock=libraryBase/constructor

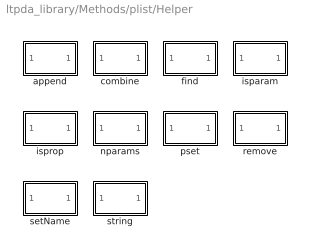
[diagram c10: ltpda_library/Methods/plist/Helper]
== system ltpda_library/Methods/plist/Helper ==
  append : Subsystem  Tag=method plist  AncestorBlock=libraryBase/function
  combine : Subsystem  Tag=method plist  AncestorBlock=libraryBase/function
  find : Subsystem  Tag=method plist  AncestorBlock=libraryBase/function
  isparam : Subsystem  Tag=method plist  AncestorBlock=libraryBase/function
  isprop : Subsystem  Tag=method plist  AncestorBlock=libraryBase/function
  nparams : Subsystem  Tag=method plist  AncestorBlock=libraryBase/function
  pset : Subsystem  Tag=method plist  AncestorBlock=libraryBase/function
  remove : Subsystem  Tag=method plist  AncestorBlock=libraryBase/function
  setName : Subsystem  Tag=method plist  AncestorBlock=libraryBase/function
  string : Subsystem  Tag=method plist  AncestorBlock=libraryBase/function

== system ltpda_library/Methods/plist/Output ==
  char : Subsystem  Tag=method plist  AncestorBlock=libraryBase/output
  display : Subsystem  Tag=method plist  AncestorBlock=libraryBase/output
  save : Subsystem  Tag=method plist  AncestorBlock=libraryBase/output

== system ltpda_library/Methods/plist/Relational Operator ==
  eq : Subsystem  Tag=method plist  AncestorBlock=libraryBase/function
  ne : Subsystem  Tag=method plist  AncestorBlock=libraryBase/function

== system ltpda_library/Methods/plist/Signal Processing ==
  resp : Subsystem  Tag=method plist  AncestorBlock=libraryBase/function

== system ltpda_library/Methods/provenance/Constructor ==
  provenance : Subsystem  Tag=method provenance  AncestorBlock=libraryBase/constructor

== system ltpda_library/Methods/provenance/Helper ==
  isprop : Subsystem  Tag=method provenance  AncestorBlock=libraryBase/function

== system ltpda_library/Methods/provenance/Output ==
  char : Subsystem  Tag=method provenance  AncestorBlock=libraryBase/output
  display : Subsystem  Tag=method provenance  AncestorBlock=libraryBase/output
  string : Subsystem  Tag=method provenance  AncestorBlock=libraryBase/output

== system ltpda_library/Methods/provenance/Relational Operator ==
  eq : Subsystem  Tag=method provenance  AncestorBlock=libraryBase/function
  ne : Subsystem  Tag=method provenance  AncestorBlock=libraryBase/function

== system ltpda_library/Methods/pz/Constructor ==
  pz : Subsystem  Tag=method pz  AncestorBlock=libraryBase/constructor

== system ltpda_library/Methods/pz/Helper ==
  isprop : Subsystem  Tag=method pz  AncestorBlock=libraryBase/function

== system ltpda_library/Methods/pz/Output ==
  char : Subsystem  Tag=method pz  AncestorBlock=libraryBase/output
  display : Subsystem  Tag=method pz  AncestorBlock=libraryBase/output
  string : Subsystem  Tag=method pz  AncestorBlock=libraryBase/output

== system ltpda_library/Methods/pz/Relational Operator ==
  eq : Subsystem  Tag=method pz  AncestorBlock=libraryBase/function
  ne : Subsystem  Tag=method pz  AncestorBlock=libraryBase/function

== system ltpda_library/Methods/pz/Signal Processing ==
  resp : Subsystem  Tag=method pz  AncestorBlock=libraryBase/function

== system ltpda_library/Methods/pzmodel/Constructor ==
  pzmodel : Subsystem  Tag=method pzmodel  AncestorBlock=libraryBase/constructor
  rebuild : Subsystem  Tag=method pzmodel  AncestorBlock=libraryBase/constructor

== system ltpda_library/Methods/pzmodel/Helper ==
  isprop : Subsystem  Tag=method pzmodel  AncestorBlock=libraryBase/function
  setIunits : Subsystem  Tag=method pzmodel  AncestorBlock=libraryBase/function
  setName : Subsystem  Tag=method pzmodel  AncestorBlock=libraryBase/function
  setOunits : Subsystem  Tag=method pzmodel  AncestorBlock=libraryBase/function
  setProperties : Subsystem  Tag=method pzmodel  AncestorBlock=libraryBase/function
  string : Subsystem  Tag=method pzmodel  AncestorBlock=libraryBase/function

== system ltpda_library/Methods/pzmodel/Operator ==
  tomfir : Subsystem  Tag=method pzmodel  AncestorBlock=libraryBase/function
  tomiir : Subsystem  Tag=method pzmodel  AncestorBlock=libraryBase/function

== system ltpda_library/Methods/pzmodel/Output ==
  char : Subsystem  Tag=method pzmodel  AncestorBlock=libraryBase/output
  display : Subsystem  Tag=method pzmodel  AncestorBlock=libraryBase/output
  save : Subsystem  Tag=method pzmodel  AncestorBlock=libraryBase/output
  type : Subsystem  Tag=method pzmodel  AncestorBlock=libraryBase/output

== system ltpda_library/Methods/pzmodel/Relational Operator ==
  eq : Subsystem  Tag=method pzmodel  AncestorBlock=libraryBase/function
  ne : Subsystem  Tag=method pzmodel  AncestorBlock=libraryBase/function

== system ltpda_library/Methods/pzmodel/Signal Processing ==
  fngen : Subsystem  Tag=method pzmodel  AncestorBlock=libraryBase/function
  resp : Subsystem  Tag=method pzmodel  AncestorBlock=libraryBase/function

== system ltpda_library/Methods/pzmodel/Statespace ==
  report : Subsystem  Tag=method pzmodel  AncestorBlock=libraryBase/function

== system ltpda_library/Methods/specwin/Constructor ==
  specwin : Subsystem  Tag=method specwin  AncestorBlock=libraryBase/constructor

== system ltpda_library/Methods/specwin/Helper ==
  isprop : Subsystem  Tag=method specwin  AncestorBlock=libraryBase/function

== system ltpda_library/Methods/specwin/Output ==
  char : Subsystem  Tag=method specwin  AncestorBlock=libraryBase/output
  display : Subsystem  Tag=method specwin  AncestorBlock=libraryBase/output
  plot : Subsystem  Tag=method specwin  AncestorBlock=libraryBase/output
  string : Subsystem  Tag=method specwin  AncestorBlock=libraryBase/output

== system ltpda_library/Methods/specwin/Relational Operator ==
  eq : Subsystem  Tag=method specwin  AncestorBlock=libraryBase/function
  ne : Subsystem  Tag=method specwin  AncestorBlock=libraryBase/function

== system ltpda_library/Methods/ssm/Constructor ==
  rebuild : Subsystem  Tag=method ssm  AncestorBlock=libraryBase/constructor
  ssm : Subsystem  Tag=method ssm  AncestorBlock=libraryBase/constructor

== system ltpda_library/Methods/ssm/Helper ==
  findParams : Subsystem  Tag=method ssm  AncestorBlock=libraryBase/function
  isprop : Subsystem  Tag=method ssm  AncestorBlock=libraryBase/function
  setName : Subsystem  Tag=method ssm  AncestorBlock=libraryBase/function
  setProperties : Subsystem  Tag=method ssm  AncestorBlock=libraryBase/function

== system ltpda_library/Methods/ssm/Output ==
  char : Subsystem  Tag=method ssm  AncestorBlock=libraryBase/output
  display : Subsystem  Tag=method ssm  AncestorBlock=libraryBase/output
  dotview : Subsystem  Tag=method ssm  AncestorBlock=libraryBase/output
  isstable : Subsystem  Tag=method ssm  AncestorBlock=libraryBase/output
  save : Subsystem  Tag=method ssm  AncestorBlock=libraryBase/output
  string : Subsystem  Tag=method ssm  AncestorBlock=libraryBase/output
  type : Subsystem  Tag=method ssm  AncestorBlock=libraryBase/output

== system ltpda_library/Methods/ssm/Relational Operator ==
  eq : Subsystem  Tag=method ssm  AncestorBlock=libraryBase/function
  ne : Subsystem  Tag=method ssm  AncestorBlock=libraryBase/function

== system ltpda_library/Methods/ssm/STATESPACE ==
  kalman : Subsystem  Tag=method ssm  AncestorBlock=libraryBase/function

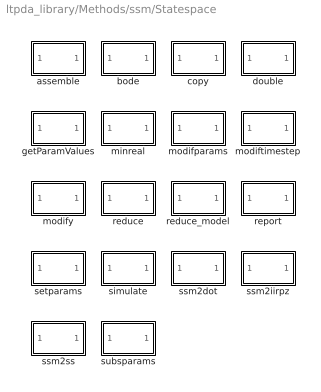
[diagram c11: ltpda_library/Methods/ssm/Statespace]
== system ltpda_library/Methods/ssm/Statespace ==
  assemble : Subsystem  Tag=method ssm  AncestorBlock=libraryBase/function
  bode : Subsystem  Tag=method ssm  AncestorBlock=libraryBase/function
  copy : Subsystem  Tag=method ssm  AncestorBlock=libraryBase/function
  double : Subsystem  Tag=method ssm  AncestorBlock=libraryBase/function
  getParamValues : Subsystem  Tag=method ssm  AncestorBlock=libraryBase/function
  minreal : Subsystem  Tag=method ssm  AncestorBlock=libraryBase/function
  modifparams : Subsystem  Tag=method ssm  AncestorBlock=libraryBase/function
  modiftimestep : Subsystem  Tag=method ssm  AncestorBlock=libraryBase/function
  modify : Subsystem  Tag=method ssm  AncestorBlock=libraryBase/function
  reduce : Subsystem  Tag=method ssm  AncestorBlock=libraryBase/function
  reduce_model : Subsystem  Tag=method ssm  AncestorBlock=libraryBase/function
  report : Subsystem  Tag=method ssm  AncestorBlock=libraryBase/function
  setparams : Subsystem  Tag=method ssm  AncestorBlock=libraryBase/function
  simulate : Subsystem  Tag=method ssm  AncestorBlock=libraryBase/function
  ssm2dot : Subsystem  Tag=method ssm  AncestorBlock=libraryBase/function
  ssm2iirpz : Subsystem  Tag=method ssm  AncestorBlock=libraryBase/function
  ssm2ss : Subsystem  Tag=method ssm  AncestorBlock=libraryBase/function
  subsparams : Subsystem  Tag=method ssm  AncestorBlock=libraryBase/function

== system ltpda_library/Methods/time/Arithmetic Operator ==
  minus : Subsystem  Tag=method time  AncestorBlock=libraryBase/function
  plus : Subsystem  Tag=method time  AncestorBlock=libraryBase/function

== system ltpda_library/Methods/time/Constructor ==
  time : Subsystem  Tag=method time  AncestorBlock=libraryBase/constructor

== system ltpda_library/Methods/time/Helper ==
  getTimezones : Subsystem  Tag=method time  AncestorBlock=libraryBase/function
  isprop : Subsystem  Tag=method time  AncestorBlock=libraryBase/function
  string : Subsystem  Tag=method time  AncestorBlock=libraryBase/function

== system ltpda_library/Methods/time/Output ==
  char : Subsystem  Tag=method time  AncestorBlock=libraryBase/output
  display : Subsystem  Tag=method time  AncestorBlock=libraryBase/output
  format : Subsystem  Tag=method time  AncestorBlock=libraryBase/output

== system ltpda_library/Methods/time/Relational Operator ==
  eq : Subsystem  Tag=method time  AncestorBlock=libraryBase/function
  ne : Subsystem  Tag=method time  AncestorBlock=libraryBase/function

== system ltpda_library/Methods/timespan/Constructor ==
  rebuild : Subsystem  Tag=method timespan  AncestorBlock=libraryBase/constructor
  timespan : Subsystem  Tag=method timespan  AncestorBlock=libraryBase/constructor

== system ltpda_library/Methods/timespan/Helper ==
  isprop : Subsystem  Tag=method timespan  AncestorBlock=libraryBase/function
  setEndT : Subsystem  Tag=method timespan  AncestorBlock=libraryBase/function
  setName : Subsystem  Tag=method timespan  AncestorBlock=libraryBase/function
  setProperties : Subsystem  Tag=method timespan  AncestorBlock=libraryBase/function
  setStartT : Subsystem  Tag=method timespan  AncestorBlock=libraryBase/function
  setTimeformat : Subsystem  Tag=method timespan  AncestorBlock=libraryBase/function
  setTimezone : Subsystem  Tag=method timespan  AncestorBlock=libraryBase/function

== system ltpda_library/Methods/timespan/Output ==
  char : Subsystem  Tag=method timespan  AncestorBlock=libraryBase/output
  display : Subsystem  Tag=method timespan  AncestorBlock=libraryBase/output
  save : Subsystem  Tag=method timespan  AncestorBlock=libraryBase/output
  string : Subsystem  Tag=method timespan  AncestorBlock=libraryBase/output
  type : Subsystem  Tag=method timespan  AncestorBlock=libraryBase/output

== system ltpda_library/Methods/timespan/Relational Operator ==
  eq : Subsystem  Tag=method timespan  AncestorBlock=libraryBase/function
  ne : Subsystem  Tag=method timespan  AncestorBlock=libraryBase/function

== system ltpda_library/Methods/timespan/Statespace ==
  report : Subsystem  Tag=method timespan  AncestorBlock=libraryBase/function

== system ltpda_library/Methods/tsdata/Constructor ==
  tsdata : Subsystem  Tag=method tsdata  AncestorBlock=libraryBase/constructor

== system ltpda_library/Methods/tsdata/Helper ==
  isprop : Subsystem  Tag=method tsdata  AncestorBlock=libraryBase/function

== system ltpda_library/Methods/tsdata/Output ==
  char : Subsystem  Tag=method tsdata  AncestorBlock=libraryBase/output
  display : Subsystem  Tag=method tsdata  AncestorBlock=libraryBase/output

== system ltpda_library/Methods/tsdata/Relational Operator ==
  eq : Subsystem  Tag=method tsdata  AncestorBlock=libraryBase/function
  ne : Subsystem  Tag=method tsdata  AncestorBlock=libraryBase/function

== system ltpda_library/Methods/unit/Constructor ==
  unit : Subsystem  Tag=method unit  AncestorBlock=libraryBase/constructor

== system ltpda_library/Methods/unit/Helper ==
  isprop : Subsystem  Tag=method unit  AncestorBlock=libraryBase/function
  string : Subsystem  Tag=method unit  AncestorBlock=libraryBase/function

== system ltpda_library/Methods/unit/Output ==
  display : Subsystem  Tag=method unit  AncestorBlock=libraryBase/output
  factor : Subsystem  Tag=method unit  AncestorBlock=libraryBase/output

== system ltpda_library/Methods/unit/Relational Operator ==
  eq : Subsystem  Tag=method unit  AncestorBlock=libraryBase/function
  ne : Subsystem  Tag=method unit  AncestorBlock=libraryBase/function

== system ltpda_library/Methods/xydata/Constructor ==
  xydata : Subsystem  Tag=method xydata  AncestorBlock=libraryBase/constructor

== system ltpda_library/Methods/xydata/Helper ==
  isprop : Subsystem  Tag=method xydata  AncestorBlock=libraryBase/function

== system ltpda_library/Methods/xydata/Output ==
  char : Subsystem  Tag=method xydata  AncestorBlock=libraryBase/output
  display : Subsystem  Tag=method xydata  AncestorBlock=libraryBase/output
